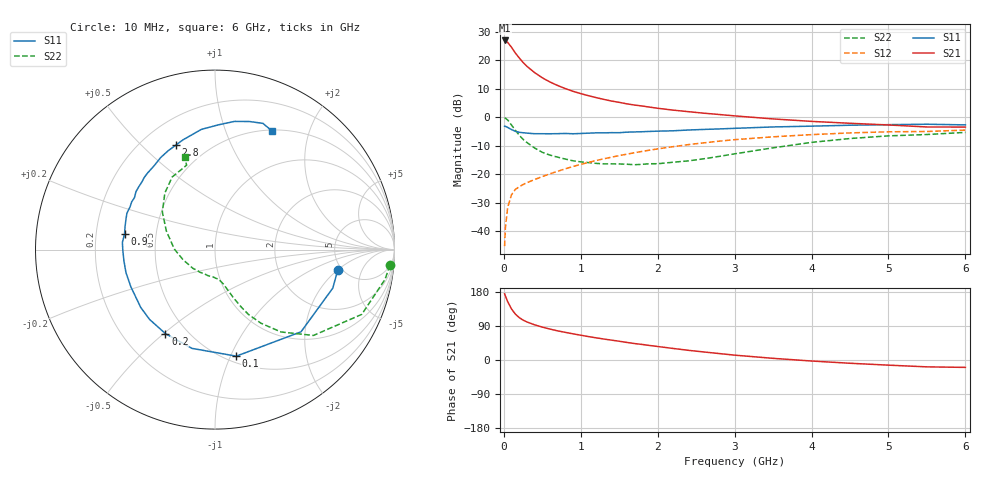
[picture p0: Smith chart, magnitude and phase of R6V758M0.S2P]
! SIEMENS Small Signal Semiconductors
! BFR193
! Si NPN RF Bipolar Junction Transistor in SOT23
! VCE = 0.75 V  IC = 8 mA
! Common Emitter S-Parameters:  May  1996
# GHz  S  MA  R  50
!  f  S11  S21  S12  S22
! GHz  MAG  ANG  MAG  ANG  MAG  ANG  MAG  ANG
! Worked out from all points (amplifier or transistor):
!   36 points, 10 MHz to 6 GHz, reference 50 ohm
!   highest |S21| = 27.0 dB at 10 MHz (marker M1)
!   |S21| within 3 dB of that: start of sweep to 114.4 MHz
!   unconditionally stable (mu >= 1): 748.5 MHz to 2.283 GHz
!   at 250 MHz: K = 0.58, MSG = 21.5 dB, |S12| = -23.7 dB
!   at 1.4 GHz: K = 1.06, MAG = 8.4 dB, |S12| = -14.1 dB
!   at 6 GHz: K = 0.99, MSG = 0.5 dB, |S12| = -4.5 dB
!   S11 on the Smith chart (normalised r, x): 10 MHz: 4.61, -2.01; 100 MHz: 0.56, -1.05; 200 MHz: 0.38, -0.51; 900 MHz: 0.33, +0.08; 2.8 GHz: 0.34, +0.64; 6 GHz: 0.51, +1.47
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0.01  0.6934 -9.4  22.35 174.7  0.0054 86.7  0.9785 -5.1
0.02  0.6905 -18.1  21.89 169.0  0.0114 83.0  0.9618 -9.9
0.05  0.663 -43.7  20.7 153.9  0.0259 71.1  0.894 -23.8
0.1  0.6054 -78.7  16.91 134.5  0.0434 58.6  0.7277 -41.1
0.15  0.5651 -103.1  13.43 121.0  0.0537 51.6  0.5879 -51.3
0.2  0.5435 -120.5  11.03 111.9  0.0598 49.0  0.4826 -58.1
0.25  0.5332 -133.1  9.166 105.3  0.0655 48.4  0.408 -62.6
0.3  0.5245 -142.1  7.837 100.4  0.0706 48.7  0.3588 -65.1
0.4  0.5126 -156.2  6.09 92.8  0.0801 50.0  0.2871 -69.1
0.5  0.5123 -165.6  4.927 86.8  0.0904 52.1  0.2413 -72.0
0.6  0.5113 -173.1  4.153 81.6  0.1011 53.7  0.2153 -74.3
0.7  0.5137 -179.5  3.607 76.9  0.1121 54.9  0.1983 -76.3
0.9  0.5114 170.2  2.851 69.0  0.1361 56.1  0.1711 -81.7
1.1  0.5239 161.3  2.388 61.8  0.1604 56.5  0.1593 -88.8
1.3  0.5298 153.3  2.055 55.3  0.1858 55.8  0.1511 -95.9
1.6  0.5459 143.8  1.716 46.3  0.2241 54.0  0.1489 -108.9
2.2  0.5767 126.2  1.332 30.5  0.3033 47.7  0.1616 -139.7
2.8  0.6218 110.5  1.115 17.0  0.3792 39.4  0.2047 -172.7
3.5  0.6742 96.4  0.933 4.4  0.4519 28.3  0.2896 159.2
4.5  0.7226 81.3  0.782 -8.6  0.5293 13.4  0.4218 131.4
5.5  0.7523 69.2  0.673 -18.1  0.5606 -0.9  0.496 108.6
6  0.7329 64.2  0.671 -19.5  0.5932 -5.2  0.5406 108.2
